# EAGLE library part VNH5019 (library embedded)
Pololu VNH5019 Motor Driver Carrier Operating voltage: 5.5 – 24 V1 Output current: 12 A continuous (30 maximum) 3V-compatible inputs PWM operation up to 20 kHz, which is ultrasonic and allows for quieter motor operation Current sense output proportional to motor current (approx. 140 mV/A; only active while H-bridge is driving) Source: VNH5019 Motor Driver Carrier
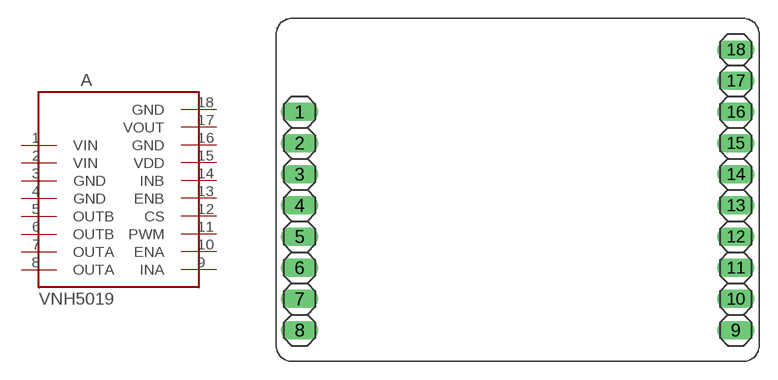
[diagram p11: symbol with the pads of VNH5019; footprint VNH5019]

Designator prefix A

## VNH5019 (DATASHEET: https://www.st.com/content/ccc/resource/technical/document/data_brief/3b/bf/c3/13/d5/b2/4c/b0/DM00101248.pdf/files/DM00101248.pdf/jcr:content/translations/en.DM00101248.pdf; DESCR: VNH5019 Motor Controller/Driver Power Management Evaluation Board; DIGIKEY_NO: 497-14839-ND; MF: Pololu; MF_PN: 1451; PURCHASE: https://www.digikey.de/product-detail/de/stmicro/EVAL-VNH5019-P1/497-14839-ND/4869482?utm_adgroup=Dev+Boards+and+Kits&mkwid=siS2m191I&pcrid=218211101233&pkw=&pmt=&pdv=c&productid=4869482&slid=&gclid=CjwKCAjw2cTmBRAVEiwA8YMgzaipRkISnCfVdTSSKNDcojFwUwpzQeKwWGZWYQUEEXtJxoFNqy7q1BoC5-sQAvD_BwE; UNIT_PRICE: 33.42)  [VNH5019]
1  VIN
2  VIN
3  GND
4  GND
5  OUTB
6  OUTB
7  OUTA
8  OUTA
9  INA
10  ENA
11  PWM
12  CS
13  ENB
14  INB
15  VDD
16  GND
17  VOUT
18  GND

## Footprint VNH5019 (pad centres in mm)
drill 1.016 long: 1 -17.78,8.89; 2 -17.78,6.35; 3 -17.78,3.81; 4 -17.78,1.27; 5 -17.78,-1.27; 6 -17.78,-3.81; 7 -17.78,-6.35; 8 -17.78,-8.89; 9 17.78,-8.89; 10 17.78,-6.35; 11 17.78,-3.81; 12 17.78,-1.27; 13 17.78,1.27; 14 17.78,3.81; 15 17.78,6.35; 16 17.78,8.89; 17 17.78,11.43; 18 17.78,13.97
